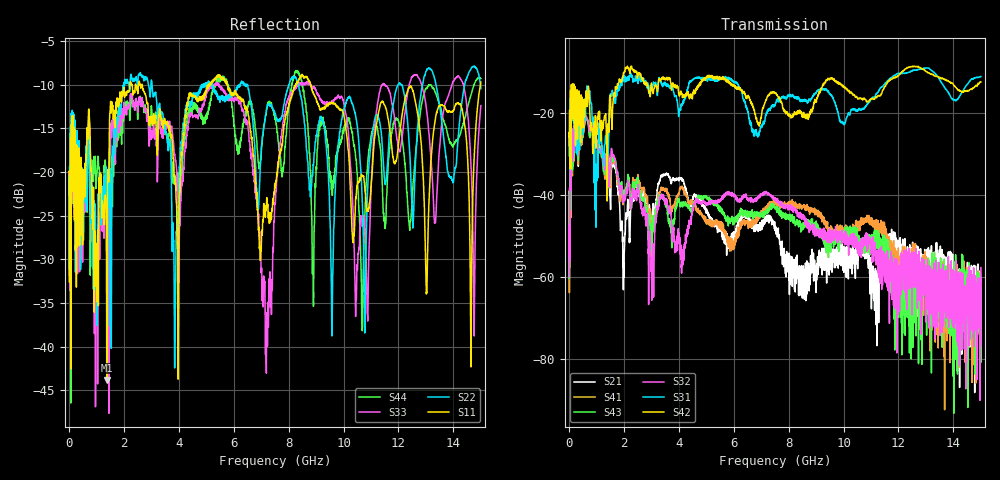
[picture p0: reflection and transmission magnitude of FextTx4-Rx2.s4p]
! FILE: N:\QM 2007\Prüfprotokolle\Highspeed\Konfektionierte Ltg\L45593-D106\D30\8216\0002\Fext\FextTx4-Rx2.s4p
# MHz S RI R 50.00
! FREQ  S11  S12  S13  S14
!  S21  S22  S23  S24
!  S31  S32  S33  S34
!  S41  S42  S43  S44
!  REAL  IMAG  REAL  IMAG  REAL  IMAG  REAL  IMAG
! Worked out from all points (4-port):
!   2999 points, 10 MHz to 15 GHz, reference 50 ohm
!   strongest paths, dB at 10 MHz, 3.755 GHz, 7.505 GHz, 11.26 GHz, 15 GHz:
!     S42: -25.8, -13.1, -15.1, -15.9, -12.5
!     S31: -24.8, -13.4, -18.3, -14.9, -11.1
!     S32: -60.0, -50.1, -40.7, -56.9, -57.8
!     S43: -39.2, -51.8, -43.2, -51.0, -62.9
!     S41: -41.1, -43.8, -41.5, -47.2, -69.2
!     S21: -44.8, -36.2, -47.9, -61.8, -66.8
!   lowest |S11| = -43.8 dB at 1.38 GHz (marker M1), VSWR 1.01, Z = 50.5 + j0.38 ohm
!   |S11| at or under -10 dB: 2.671 GHz to 5.107 GHz (2.436 GHz wide, 62.6 % of centre); 5.776 GHz to 8.261 GHz (2.485 GHz wide, 35.4 % of centre); 8.798 GHz to 14.98 GHz (6.184 GHz wide, 52 % of centre)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
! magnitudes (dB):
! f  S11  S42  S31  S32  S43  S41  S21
! 10 MHz  -19.9  -25.8  -24.8  -60.0  -39.2  -41.1  -44.8
! 210 MHz  -21.8  -23.6  -21.2  -23.4  -24.4  -24.4  -24.0
! 1.38 GHz  -43.8  -28.7  -25.9  -30.5  -30.0  -29.9  -31.5
! 3.045 GHz  -14.6  -14.6  -13.8  -54.5  -47.2  -49.3  -44.3
! 7.205 GHz  -22.9  -16.5  -20.1  -39.4  -44.6  -43.5  -46.5
! 8.325 GHz  -9.8  -19.6  -16.2  -44.8  -46.7  -43.3  -58.4
! 15 GHz  -9.7  -12.5  -11.1  -57.8  -62.9  -69.2  -66.8
